FUNCTION_BLOCK Example11_readxbotposition //>= 1 xbot
VAR_INPUT
	Execute : BOOL;
END_VAR
VAR_OUTPUT
	posX : REAL;
	posY : REAL;
	posZ : REAL;
	posRx : REAL;
	posRy : REAL;
	posRz : REAL;
END_VAR
VAR_IN_OUT
	PM_Controller : PMControllerType;	// the planar motor controller to use
END_VAR
VAR
	PMC_ReadXbotPos1 : PMC_ReadXbotPos;
END_VAR

//>= 1 xbot

PMC_ReadXbotPos1(Enable := Execute,XbotID := 1,PosX => posX,PosY => posY,PosZ => posZ,PosRx => posRx,PosRy => posRy,PosRz => posRz,PM_Controller := PM_Controller);

END_FUNCTION_BLOCK
